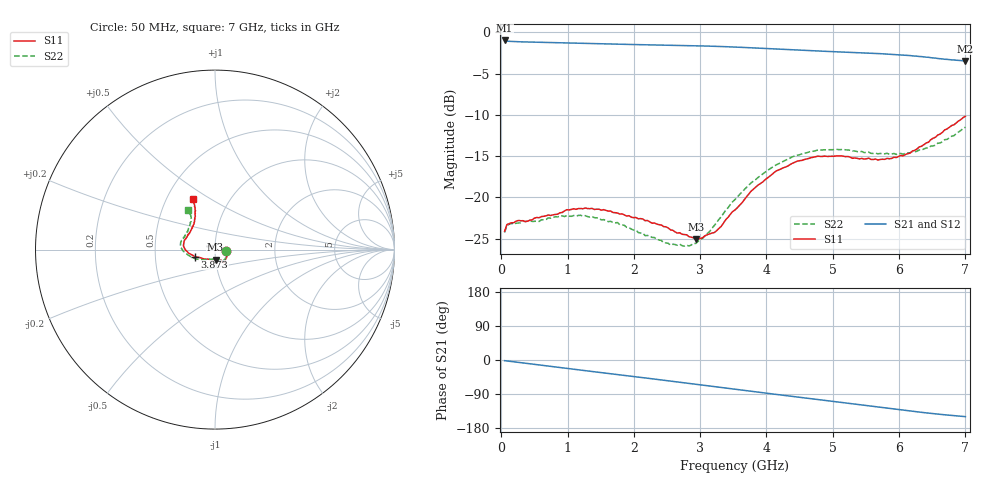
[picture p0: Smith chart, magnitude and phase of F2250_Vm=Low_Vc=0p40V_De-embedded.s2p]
! Integrated Device Technology
! Corporate Headquarters
! 6024 Silver Creek Valley Road
! San Jose, CA 95138  USA
! Phone:  1-408-284-8200
! Toll Free:  1-800-223-1366
! Webpage:  http://www.idt.com/
! Timing and RF Division
! 515 Groton Road, Suite 102
! Westford, MA 01886-6024
! Device:  F2250
! Description: Voltage Variable RF Attenuator
! Frequency:  50.0 -  6000.00 MHz
! Package:  3x3 mm Thin QFN Plastic Package: 16 pin
! Ports:  2 RF, 3 DC
!  Pin  1  = GND
!  Pin  2  = NC
!  Pin  3  = RF1  = Port 1
!  Pin  4  = NC
!  Pin  5  = GND
!  Pin  6  = GND
!  Pin  7  = GND
!  Pin  8  = GND
!  Pin  9  = NC
!  Pin 10  = RF2  = Port 2
!  Pin 11  = NC
!  Pin 12  = GND
!  Pin 13  = GND
!  Pin 14  = VCNTRL
!  Pin 15  = VDD
!  Pin 16  = VMODE
! Vcntrl:  0.400 Volts
! Vmode:  +0.000 Volts
! Vdd:  +3.30  Volts
! Current:  1.123 mA
! Data:  The device was measured on a the F2250 evaluation board which has
!  individual transmission lines to the RF pins.  Data was collected
!  using a calibrated network analyzer.  The evaluation board was
!  de-embedded using a TRL calibration technique.
!  The reference plane is the edge of the package pin.
! Misc:  SN 10
!  Action Tracker AT0258
! Date Measured:  2014-11-26
! Date:  2015-10-15  MJV
! Note:
!  Integrated Device Technology supplies this data as a sample of measured
!  data at the package pin for this product.  Your particular data for this
!  product may vary.
!  Data was taken at 25 degrees C.
!  Integrated Device Technology reserves the right to change this data at anytime.
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# GHz S dB R 50
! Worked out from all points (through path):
!   201 points, 50 MHz to 7 GHz, reference 50 ohm
!   highest |S21| = -0.99 dB at 50 MHz (marker M1); lowest = -3.5 dB at 7 GHz (marker M2)
!   group delay of S21, straight-line fit = 60 ps
!   lowest |S11| = -25.1 dB at 2.934 GHz (marker M3), VSWR 1.12, Z = 50 - j5.58 ohm
!   |S11| at or under -10 dB: start of sweep to end of sweep
!   |S22| runs from -25.9 to -11.5 dB; largest |S21 - S12| = 0.0004
!   S11 on the Smith chart (normalised r, x): 50 MHz: 1.13, -0.02; 3.873 GHz: 0.80, -0.06; 7 GHz: 0.67, +0.42
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0.05  -24.10 -8.8  -0.99 -1.8  -0.99 -1.8  -24.25 -9.4
0.08475  -23.30 -8.7  -1.07 -2.5  -1.07 -2.5  -23.39 -8.7
0.15425  -23.08 -10.9  -1.11 -4.0  -1.11 -4.0  -23.16 -10.5
0.6755  -22.23 -33.7  -1.24 -15.4  -1.24 -15.4  -22.66 -35.0
0.884  -21.86 -43.0  -1.28 -20.0  -1.28 -20.0  -22.25 -45.2
1.2315  -21.38 -52.9  -1.36 -27.4  -1.36 -27.4  -22.25 -57.9
1.75275  -21.88 -59.6  -1.45 -38.4  -1.45 -38.4  -23.04 -65.7
2.37825  -23.30 -60.8  -1.54 -51.8  -1.54 -51.8  -25.16 -69.2
2.552  -23.93 -64.6  -1.57 -55.6  -1.56 -55.6  -25.77 -74.9
2.83  -24.75 -78.5  -1.62 -61.7  -1.61 -61.7  -25.89 -93.0
2.93425  -25.07 -86.7  -1.64 -64.0  -1.63 -64.0  -25.58 -101.2
3.21225  -24.26 -115.5  -1.70 -70.2  -1.70 -70.2  -23.40 -126.0
3.525  -21.52 -143.4  -1.79 -77.1  -1.79 -77.1  -20.26 -145.0
3.8725  -18.51 -160.9  -1.92 -84.8  -1.92 -84.8  -17.59 -160.5
4.1505  -16.78 -171.1  -2.04 -90.9  -2.03 -90.9  -16.04 -170.5
4.4285  -15.74 -178.9  -2.14 -96.9  -2.14 -96.9  -14.97 -177.7
4.7065  -15.13 174.3  -2.25 -102.9  -2.25 -102.9  -14.41 176.2
5.15825  -15.01 163.5  -2.41 -112.6  -2.40 -112.6  -14.17 166.9
5.85325  -15.32 140.1  -2.65 -127.6  -2.65 -127.6  -14.77 151.6
6.166  -14.64 129.0  -2.82 -134.4  -2.82 -134.4  -14.60 142.7
6.444  -13.31 120.4  -3.03 -140.2  -3.03 -140.2  -14.01 133.3
7  -10.18 113.8  -3.47 -149.5  -3.48 -149.5  -11.50 123.9
